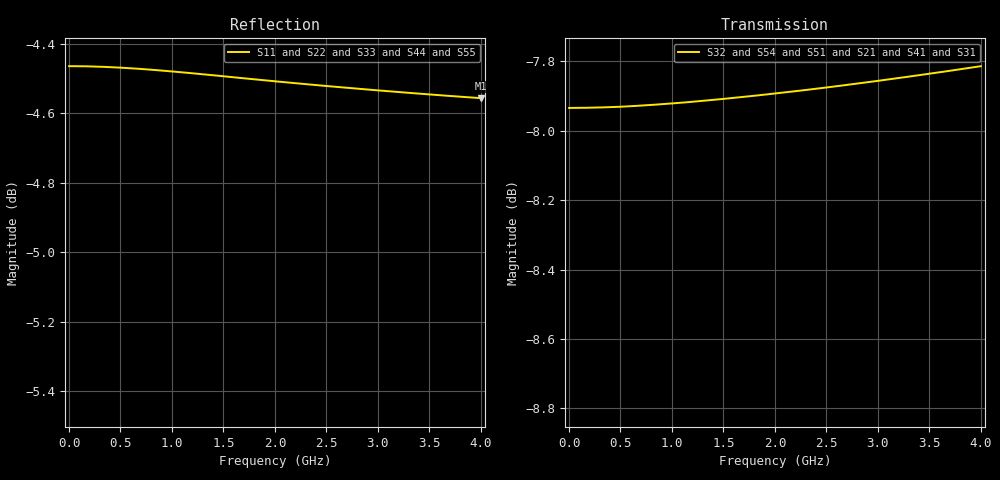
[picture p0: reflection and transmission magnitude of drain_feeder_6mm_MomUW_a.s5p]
! Created Thu Sep 17 15:56:28 2015
# ghz S ma R 50
! 5 Port Network Data from data block
! freq  magS11  angS11  magS12  angS12  magS13  angS13  magS14  angS14
!  magS15  angS15
!  magS21  angS21  magS22  angS22  magS23  angS23
!  magS24  angS24  magS25  angS25
!  magS31  angS31  magS32  angS32
!  magS33  angS33  magS34  angS34  magS35  angS35
!  magS41  angS41
!  magS42  angS42  magS43  angS43  magS44  angS44  magS45  angS45
!  magS51  angS51  magS52  angS52  magS53  angS53  magS54  angS54
!  magS55  angS55
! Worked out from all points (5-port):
!   23 points, 1 MHz to 4 GHz, reference 50 ohm
!   strongest paths, dB at 1 MHz, 500.9 MHz, 1.501 GHz, 2.5 GHz, 4 GHz:
!     S32: -7.9, -7.9, -7.9, -7.9, -7.8
!     S54: -7.9, -7.9, -7.9, -7.9, -7.8
!     S51: -8.0, -8.0, -8.0, -8.0, -8.0
!     S21: -8.0, -8.0, -8.0, -8.0, -8.0
!     S41: -8.0, -8.0, -8.0, -8.0, -8.0
!     S31: -8.0, -8.0, -8.0, -8.0, -8.0
!   lowest |S11| = -4.6 dB at 4 GHz (marker M1), VSWR 3.90, Z = 12.8 + j1.01 ohm
!   |S11| at or under -10 dB: nowhere
